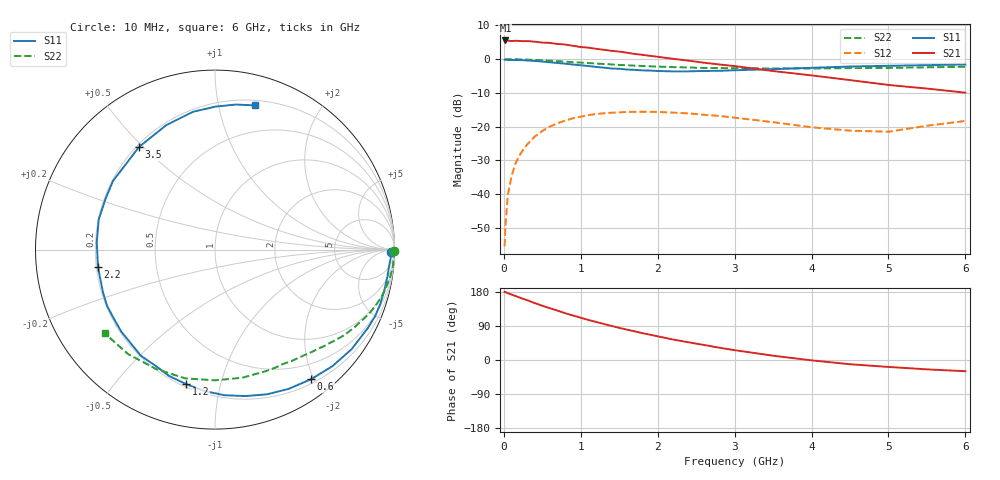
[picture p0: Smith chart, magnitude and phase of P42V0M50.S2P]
! SIEMENS Small Signal Semiconductors
! BFP182
! Si NPN RF Bipolar Junction Transistor in SOT143
! VCE = 2 V  IC = 0.5 mA
! Common Emitter S-Parameters:  March  1996
# GHz  S  MA  R  50
!  f  S11  S21  S12  S22
! GHz  MAG  ANG  MAG  ANG  MAG  ANG  MAG  ANG
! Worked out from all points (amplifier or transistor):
!   36 points, 10 MHz to 6 GHz, reference 50 ohm
!   highest |S21| = 5.5 dB at 20 MHz (marker M1)
!   |S21| within 3 dB of that: start of sweep to 1.375 GHz
!   unconditionally stable (mu >= 1): 2.95 GHz to end of sweep
!   at 250 MHz: K = 0.09, MSG = 16.1 dB, |S12| = -26.9 dB
!   at 1.4 GHz: K = 0.50, MSG = 9.2 dB, |S12| = -15.9 dB
!   at 6 GHz: K = 1.22, MAG = 1.3 dB, |S12| = -18.3 dB
!   S11 on the Smith chart (normalised r, x): 10 MHz: 63, -53; 600 MHz: 0.26, -1.96; 1.2 GHz: 0.22, -0.79; 2.2 GHz: 0.21, -0.07; 3.5 GHz: 0.21, +0.49; 6 GHz: 0.24, +1.28
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0.01  0.9815 -0.9  1.855 179.7  0.0017 84.9  0.9994 -0.3
0.02  0.9828 -1.7  1.893 179.3  0.0033 83.0  0.9999 -0.7
0.05  0.9757 -4.6  1.884 176.4  0.0094 88.7  0.9989 -1.6
0.1  0.9722 -9.0  1.853 172.7  0.0185 83.1  0.9945 -3.2
0.15  0.9702 -13.6  1.874 169.0  0.0282 80.7  0.996 -5.0
0.3  0.957 -27.2  1.854 158.2  0.0541 72.2  0.9849 -9.8
0.4  0.942 -36.1  1.816 150.3  0.0711 66.5  0.9749 -13.0
0.6  0.8991 -53.4  1.74 136.5  0.1005 55.4  0.9492 -18.9
0.8  0.8565 -70.3  1.645 123.4  0.1235 45.0  0.9186 -24.3
1.1  0.7905 -94.2  1.479 105.6  0.1483 31.8  0.8751 -31.4
1.2  0.767 -102.0  1.423 100.4  0.1542 27.3  0.8623 -33.7
1.4  0.7272 -117.1  1.328 89.9  0.161 19.9  0.8353 -37.6
1.6  0.7023 -131.7  1.247 80.1  0.1657 13.4  0.8133 -41.3
1.9  0.678 -152.5  1.12 66.8  0.1663 4.6  0.7841 -46.7
2.2  0.6593 -171.4  1.012 54.0  0.1615 -2.6  0.763 -51.9
2.8  0.672 155.4  0.835 32.5  0.1444 -14.0  0.7385 -63.0
3.5  0.7115 126.5  0.667 11.3  0.1166 -20.0  0.73 -78.0
4  0.7447 111.4  0.575 -0.9  0.098 -17.0  0.7282 -90.1
4.5  0.7778 99.0  0.49 -11.2  0.0874 -10.0  0.7364 -103.1
5  0.7966 89.8  0.415 -18.3  0.0842 4.7  0.7421 -116.3
5.5  0.8165 81.8  0.367 -24.7  0.1032 12.2  0.7572 -129.8
6  0.8334 74.6  0.319 -29.6  0.1216 14.1  0.7713 -142.8
